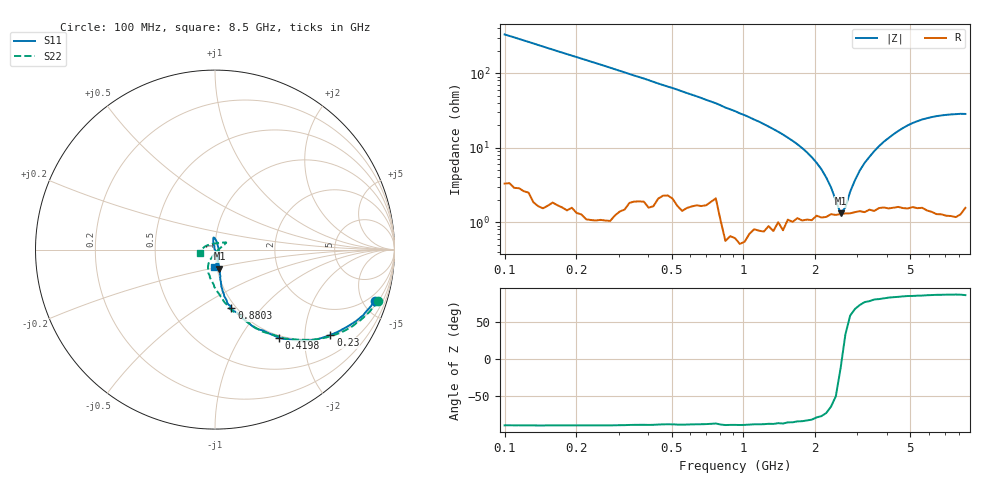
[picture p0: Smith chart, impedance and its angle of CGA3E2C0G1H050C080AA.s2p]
! S-parameter Generated by TDK Corporation
! Copyright(C) 2015 TDK Corporation.
! All Rights Reserved.
! TDK P/N: CGA3E2C0G1H050C080AA (Multilayer Ceramic Chip Capacitors)
! Property: C=5pF
! Size(LxWxT): 1.6x0.8x0.8mm, 0.063x0.031x0.031inches
! Model Type: s2p (Touchstone File Format Version 1.0)
! Frequency: DC=Yes Start=100MHz Stop=8500MHz 98points Log-sweep
! Note:
! Model Generated on Jun. 23, 2015
! Hash(MD5):
! Port Assignments:
!  1 ---| |--- 2
! Applicable Conditions:
!  Temperature = 25 degC
!  DC Bias Voltage = 0 V
!  Small Signal Operation
! Terms and conditions regarding TDK Simulation Models
! (1)This simulation model is being provided solely for informational purposes. Please refer to the specifications of the products in terms of detailed characteristics of such products.
! (2)In no event shall TDK Corporation of any of its subsidiaries be liable for any loss or damage arising, directly or indirectly,
!  From any information contained in this simulation model, including, but not limited to loss or damages arising from any inaccuracies, omissions or errors in connection with such information.
! (3)Any and all copyrights on this simulation model are owned by TDK Corporation.
!  Duplication or redistribution of this simulation model without prior written permission from TDK Corporation is prohibited.
! (4)This simulation model is subject to any modification or change without any prior notice.
! (5)Neither TDK Corporation nor any of its subsidiaries shall make any warranty, express or implied,
!  Including but not limited to the correctness, implied warranties of merchantability and fitness for a particular purpose with respect to this simulation models.
! (6)The use of this simulation model shall be deemed to have consented to the terms and conditions hereof.
# MHz S MA R 50
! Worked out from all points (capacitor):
!   97 points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, 100 MHz to 8.5 GHz, reference 50 ohm
!   read as one part in series: C = 4.81 pF near 100 MHz
!   lowest |Z| = 1.32 ohm at 2.552 GHz (marker M1)
!   series resonance near 2.581 GHz, so ESL is about 790 pH
!   S11 on the Smith chart (normalised r, x): 100 MHz: 1.30, -6.13; 230 MHz: 1.02, -2.69; 419.8 MHz: 0.97, -1.50; 880.3 MHz: 0.95, -0.70; 8.5 GHz: 0.97, -0.19
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100  0.9372 -17.8  0.286 72.0  0.2858 71.9  0.9516 -17.4
230.0202  0.7993 -36.5  0.5611 53.7  0.5599 53.7  0.8134 -35.9
419.7991  0.6055 -54.0  0.7747 35.5  0.7749 35.4  0.6082 -53.3
880.2608  0.3387 -74.3  0.9244 15.5  0.9237 15.5  0.3449 -75.3
1533.871  0.2019 -80.0  0.9603 3.5  0.9611 3.7  0.1983 -91.7
2551.925  0.1082 -77.0  0.9719 -5.9  0.9718 -5.8  0.1114 -110.6
2931.989  0.0821 -76.1  0.9729 -8.6  0.9731 -8.5  0.08459 -114.9
3368.656  0.04921 -74.8  0.9751 -11.4  0.9744 -11.4  0.05399 -112.9
3695.327  0.02396 -78.1  0.9745 -13.5  0.9739 -13.4  0.02853 -100.3
3870.357  0.007791 -60.2  0.9747 -14.5  0.9736 -14.5  0.01893 -82.5
4053.677  0.004757 129.6  0.9743 -15.6  0.9733 -15.5  0.01507 -32.7
4245.68  0.01914 102.8  0.9738 -16.7  0.9727 -16.7  0.02199 6.8
4446.777  0.03182 104.9  0.9725 -18.0  0.9703 -17.8  0.03545 19.9
4657.399  0.04506 102.2  0.9709 -19.2  0.9721 -19.1  0.0473 26.6
5109.044  0.06308 98.7  0.9693 -21.8  0.9684 -21.7  0.06787 30.9
5869.945  0.06425 92.1  0.9695 -25.9  0.9649 -25.7  0.06855 35.5
6439.175  0.04409 76.5  0.9679 -28.9  0.9659 -28.7  0.04967 52.2
6744.168  0.02702 54.8  0.9662 -30.4  0.9687 -30.4  0.03803 70.5
7063.606  0.02087 -2.0  0.9655 -32.3  0.965 -32.0  0.03518 105.1
7398.175  0.0355 -48.8  0.9661 -33.9  0.9667 -33.9  0.04201 137.3
7748.59  0.05647 -70.3  0.963 -35.9  0.9652 -35.8  0.05745 161.0
8500  0.09713 -94.4  0.9594 -39.9  0.9583 -39.7  0.08471 -165.6
